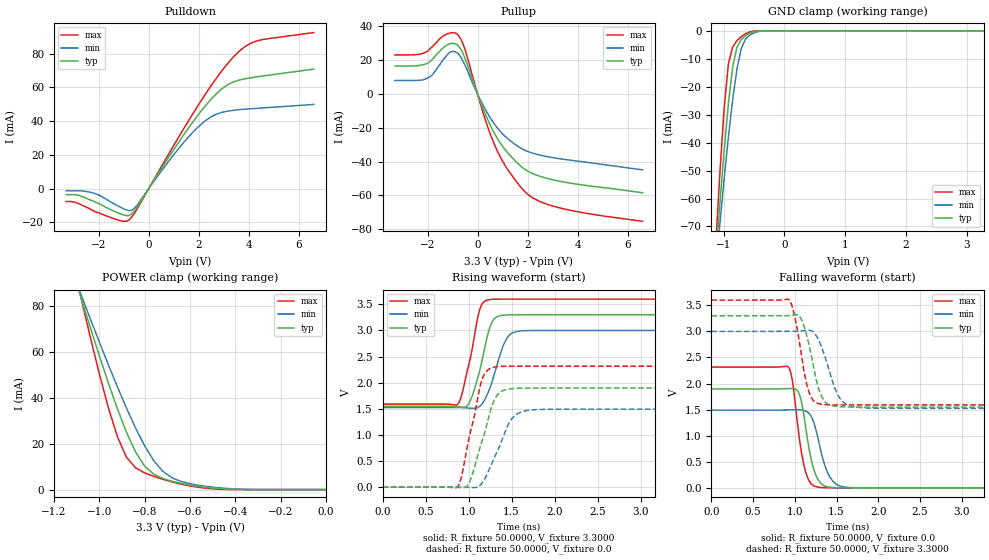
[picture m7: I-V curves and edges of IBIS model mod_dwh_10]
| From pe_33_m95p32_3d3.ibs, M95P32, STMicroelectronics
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|   Model mod_dwh_10
[Model]   mod_dwh_10
Model_type I/O
Polarity   Non-Inverting
Vinl   =   1.000V
Vinh   =   2.300V
Vmeas  =   1.650V
Cref   =   30pF
C_comp   1.607pF   1.535pF   1.683pF
[Model Spec]
Vinl   1.000V  0.900V  1.080V  | <- for Vcc = 3.3V, 3.0V, 3.6V
Vinh   2.300V  2.100V  2.520V  | <- for Vcc = 3.3V, 3.0V, 3.6V
Vmeas  1.650V  1.500V  1.800V  | <- for Vcc = 3.3V, 3.0V, 3.6V
[Temperature Range]   25.0000   0.1050k   -40.0000
[Voltage Range]   3.3000V   3.0000V   3.6000V
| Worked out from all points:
|   slope of the pulldown table from 0 to 0.495 V, typ, clamps not added: 42.6 ohm
|   slope of the pullup table from 0 to 0.495 V, typ, clamps not added: 27.6 ohm
|   GND clamp passes 1 mA (typ) near -0.58 V on its own axis
|   POWER clamp passes 1 mA (typ) near -0.53 V on its own axis
|   rising waveform, R_fixture 50.0000, V_fixture 3.3000: 20-80 % time 156ps typ, 173ps min, 148ps max; typ from 1.55 V to 3.3 V
|   rising waveform, R_fixture 50.0000, V_fixture 0.0: 20-80 % time 196ps typ, 232ps min, 174ps max; typ from 0 V to 1.9 V
|   falling waveform, R_fixture 50.0000, V_fixture 0.0: 20-80 % time 127ps typ, 153ps min, 118ps max; typ from 1.9 V to 0 V
|   falling waveform, R_fixture 50.0000, V_fixture 3.3000: 20-80 % time 148ps typ, 185ps min, 131ps max; typ from 3.3 V to 1.55 V
[Pulldown]
|Voltage   I(typ)   I(min)   I(max)
-3.3V     -3.6mA     -1.32mA    -7.7mA
-2.9V     -3.7mA     -1.32mA    -8.34mA
-2.2V     -7.5mA     -2.7mA     -13.3mA
-1.2V     -14.6mA    -10.5mA    -18.8mA
-800mV    -16.01mA   -13.02mA   -18.69mA
-500mV    -11.75mA   -10.47mA   -12.96mA
1V        23.15mA    20.08mA    25.61mA
2V        44.19mA    36.88mA    49.93mA
2.8V      57.58mA    44.65mA    67.43mA
3.5V      63.91mA    46.64mA    79.85mA
4.4V      66.5mA     47.7mA     87.91mA
6.6V      70.9mA     49.94mA    92.6mA
[Pullup]
|Voltage   I(typ)   I(min)   I(max)
-3.3V     16.6mA     8.02mA     23.18mA
-2.1V     17.69mA    8.788mA    24.57mA
-1.8V     20.64mA    11.45mA    28.17mA
-1.1V     29.8mA     24.81mA    36.14mA
-800mV    29.14mA    24.26mA    35.36mA
-500mV    21.02mA    17.03mA    26.58mA
200mV     -7.817mA   -5.983mA   -10.07mA
700mV     -23.89mA   -18.2mA    -30.68mA
1.2V      -34.67mA   -26.28mA   -44.52mA
1.9V      -44.59mA   -33.29mA   -57.84mA
3.3V      -51.61mA   -38.3mA    -67.42mA
6.6V      -58.4mA    -44.87mA   -75.3mA
[GND_clamp]
|Voltage   I(typ)   I(min)   I(max)
-3.3V     -807.6mA   -672mA     -1.053A
-1.13V    -81.94mA   -85.75mA   -76.94mA
-1.06V    -61.58mA   -68.96mA   -50.51mA
-990mV    -42.58mA   -52.9mA    -27.53mA
-920mV    -25.81mA   -37.91mA   -11.64mA
-850mV    -12.88mA   -24.52mA   -5.709mA
-780mV    -5.82mA    -13.61mA   -3.523mA
-710mV    -3.106mA   -6.377mA   -2.091mA
-640mV    -1.742mA   -2.986mA   -1.046mA
-500mV    -309.6uA   -721.8uA   -69.16uA
-290mV    -791nA     -10.61uA   -17.06nA
3.28V     561.4pA    18.21uA    173.1pA
[POWER_clamp]
|Voltage   I(typ)   I(min)   I(max)
-3.28V    853.2mA    705.5mA    1.123A
-1.08V    83.64mA    85.1mA     83.66mA
-1V       58.53mA    64.51mA    50.75mA
-960mV    46.59mA    54.53mA    35.87mA
-920mV    35.3mA     44.85mA    23.13mA
-880mV    25.04mA    35.59mA    14.12mA
-840mV    16.42mA    26.93mA    9.512mA
-800mV    10.26mA    19.14mA    7.302mA
-720mV    4.876mA    8.001mA    4.493mA
-640mV    2.758mA    3.578mA    2.397mA
-400mV    94.29uA    284.7uA    12.64uA
0V        840.7pA    17.31nA    345.8pA
[Ramp]
| variable   typ   min   max
dV/dt_r   1.1383/0.2199n   0.9181/0.2519n   1.3897/0.1890n
dV/dt_f   1.0516/0.1761n   0.8992/0.2300n   1.2059/0.1614n
R_load = 50.0000
[Rising Waveform]
R_fixture= 50.0000
V_fixture= 3.3000
V_fixture_min= 3.0000
V_fixture_max= 3.6000
|time   V(typ)   V(min)   V(max)
0s        1.547V     1.524V     1.59V
872ps     1.541V     1.525V     1.584V
920ps     1.533V     1.522V     1.766V
1.032ns   1.702V     1.511V     2.561V
1.128ns   2.222V     1.546V     3.392V
1.224ns   2.927V     1.799V     3.585V
1.288ns   3.2V       2.098V     3.597V
1.416ns   3.294V     2.759V     3.6V
1.576ns   3.3V       2.985V     3.6V
6ns       3.3V       3V         3.6V
[Rising Waveform]
R_fixture= 50.0000
V_fixture= 0.0
V_fixture_min= 0.0
V_fixture_max= 0.0
|time   V(typ)   V(min)   V(max)
0s        6.853nV    730.9nV    1.212nV
880ps     -4.601mV   520uV      22.21mV
928ps     -10.8mV    -684.4uV   276.5mV
1.008ns   88.88mV    -5.374mV   964.7mV
1.152ns   859.3mV    68.71mV    2.038V
1.216ns   1.219V     252mV      2.231V
1.296ns   1.661V     553.2mV    2.297V
1.504ns   1.886V     1.311V     2.316V
1.712ns   1.896V     1.475V     2.316V
6ns       1.897V     1.493V     2.316V
[Falling Waveform]
R_fixture= 50.0000
V_fixture= 0.0
V_fixture_min= 0.0
V_fixture_max= 0.0
|time   V(typ)   V(min)   V(max)
0s        1.897V     1.493V     2.316V
920ps     1.904V     1.495V     2.321V
968ps     1.905V     1.497V     2.075V
1.048ns   1.82V      1.499V     1.02V
1.112ns   1.356V     1.483V     414mV
1.192ns   573.2mV    1.381V     84.33mV
1.256ns   229.4mV    1.093V     21.45mV
1.4ns     17.32mV    267.8mV    1.5mV
1.592ns   1.056mV    17.33mV    67.99uV
6ns       1.915uV    2.763uV    2.005uV
[Falling Waveform]
R_fixture= 50.0000
V_fixture= 3.3000
V_fixture_min= 3.0000
V_fixture_max= 3.6000
|time   V(typ)   V(min)   V(max)
0s        3.3V       3V         3.6V
928ps     3.303V     2.999V     3.611V
992ps     3.316V     3V         3.331V
1.088ns   3.199V     3.009V     2.451V
1.184ns   2.641V     3.021V     1.777V
1.296ns   1.851V     2.796V     1.61V
1.376ns   1.632V     2.443V     1.595V
1.52ns    1.558V     1.77V      1.591V
1.712ns   1.548V     1.553V     1.59V
6ns       1.547V     1.524V     1.59V
